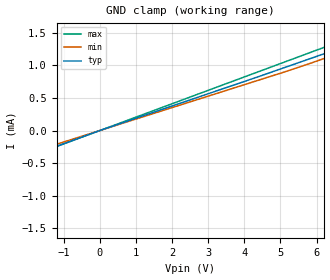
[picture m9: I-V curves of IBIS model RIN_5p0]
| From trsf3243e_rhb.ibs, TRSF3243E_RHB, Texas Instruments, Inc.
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[Model]   RIN_5p0
Model_type   Input
Vinl = 0.8
Vinh = 2.4
|   typ   min   max
C_comp   1.05pF   0.83pF   1.39pF
[Voltage Range]   5   4.5   5.5
[Temperature Range]   27   110   -40
[Power Clamp Reference]   5   4.5   5.5
[GND Clamp Reference]   0   0   0
[GND Clamp]
|   Voltage   I(typ)   I(min)   I(max)
-25V      -5.17mA    -4.824mA   -5.654mA
-11.69V   -2.401mA   -2.239mA   -2.628mA
-6.141V   -1.246mA   -1.16mA    -1.365mA
-1.35V    -273.4uA   -237.5uA   -277.7uA
-35.35mV  -6.566uA   -6.122uA   -7.186uA
5.176V    979.6uA    911.6uA    1.065mA
7.701V    1.479mA    1.394mA    1.603mA
8.039V    1.549mA    1.459mA    1.679mA
8.872V    1.722mA    1.62mA     1.868mA
25V       5.073mA    4.75mA     5.53mA
